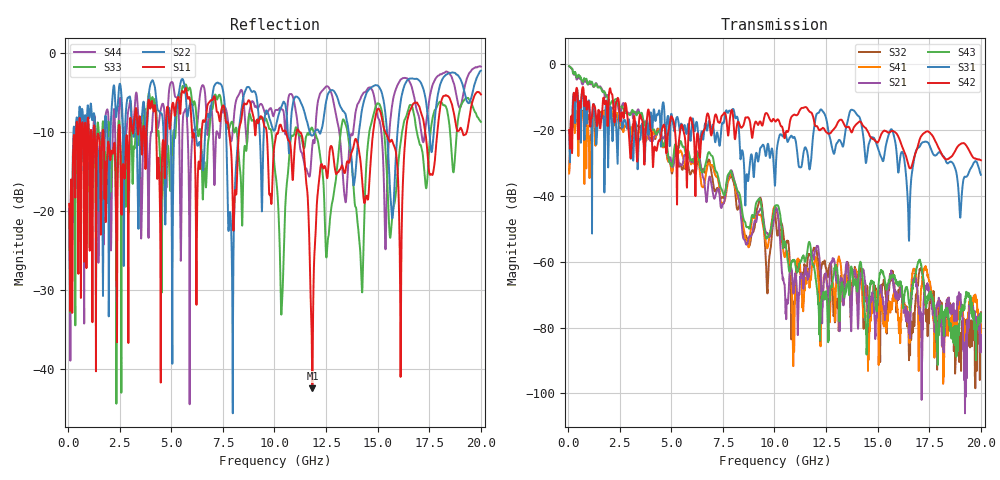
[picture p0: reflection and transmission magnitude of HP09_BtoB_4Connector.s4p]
# MHz S MA R 50.00
! FREQ  S11  S12  S13  S14
!  S21  S22  S23  S24
!  S31  S32  S33  S34
!  S41  S42  S43  S44
!  MAG  ANG  MAG  ANG  MAG  ANG  MAG  ANG
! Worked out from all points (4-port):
!   1996 points, 50 MHz to 20 GHz, reference 50 ohm
!   strongest paths, dB at 50 MHz, 5.04 GHz, 10.03 GHz, 15.02 GHz, 20 GHz:
!     S42: -20.0, -16.2, -17.4, -23.7, -29.2
!     S31: -20.2, -16.2, -36.6, -25.7, -33.6
!     S43: -0.6, -30.9, -43.2, -69.0, -77.9
!     S21: -0.7, -31.1, -44.7, -69.8, -82.3
!     S41: -33.2, -32.6, -43.2, -76.1, -83.0
!     S32: -32.3, -33.2, -45.5, -71.8, -75.3
!   lowest |S11| = -42.5 dB at 11.84 GHz (marker M1), VSWR 1.02, Z = 49.4 + j0.381 ohm
!   |S11| at or under -10 dB: 1.714 GHz to 2.445 GHz (731 MHz wide, 35.2 % of centre); 11.2 GHz to 14.78 GHz (3.584 GHz wide, 27.6 % of centre); 15.36 GHz to 16.37 GHz (1.008 GHz wide, 6.35 % of centre)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
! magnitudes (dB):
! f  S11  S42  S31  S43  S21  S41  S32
! 50 MHz  -19.1  -20.0  -20.2  -0.6  -0.7  -33.2  -32.3
! 4.38 GHz  -13.3  -23.4  -14.7  -20.4  -20.6  -19.7  -19.7
! 7.95 GHz  -15.8  -14.1  -13.8  -33.7  -32.7  -33.6  -34.5
! 8.76 GHz  -6.0  -16.5  -33.5  -49.9  -52.6  -55.4  -55.3
! 10.35 GHz  -9.5  -18.9  -21.6  -50.3  -61.9  -53.5  -48.5
! 11.84 GHz  -42.5  -15.4  -23.8  -60.7  -57.9  -60.8  -57.2
! 20 GHz  -5.3  -29.2  -33.6  -77.9  -82.3  -83.0  -75.3
